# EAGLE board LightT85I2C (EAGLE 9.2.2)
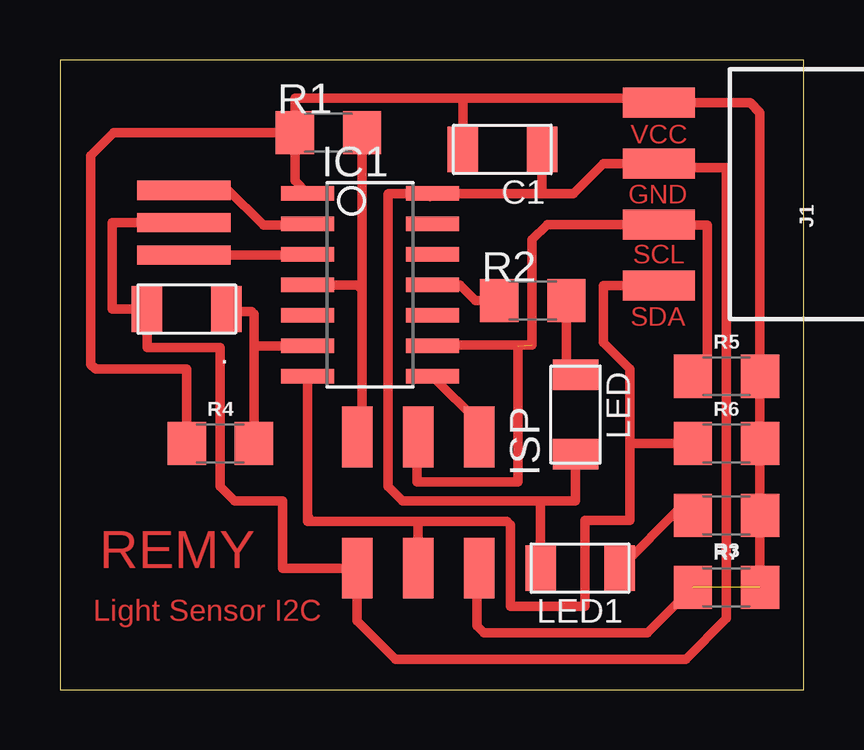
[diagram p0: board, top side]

Size 31 x 26.26 mm. Coordinates in mm from the lower left corner, seen from the top.
Outline: 0,0 31,0 31,26.26 0,26.26 0,0
Copper layers (1*16): Top 0.035mm / dielectric 1.5mm / Bottom 0.035mm
Design rules "default *": minimum track width 0.4mm, minimum drill 0.4mm, track to track 0.3mm, track to pad 0.3mm, pad to pad 0.3mm, via to via 6mil, smd to smd 0.3mm, copper to edge 40mil, drill to drill 6mil, minimum pad ring 10mil, minimum via ring 8mil, stop-mask expansion 4mil, vias tented up to drill 0mil, thermal gap 10mil

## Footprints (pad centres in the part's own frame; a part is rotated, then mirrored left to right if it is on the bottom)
LED1206FAB = smd 1.27 x 1.905: 1 -1.651,0; 2 1.651,0
C1206FAB = smd 1.27 x 1.905: 1 -1.651,0; 2 1.651,0
SOIC14 = smd 0.61 x 2.21: 1 -3.81,-2.603; 2 -2.54,-2.603; 3 -1.27,-2.603; 4 0,-2.603; 5 1.27,-2.603; 6 2.54,-2.603; 7 3.81,-2.603; 8 3.81,2.603; 9 2.54,2.603; 10 1.27,2.603; 11 0,2.603; 12 -1.27,2.603; 13 -2.54,2.603; 14 -3.81,2.603
2X03SMD = smd 2.54 x 1.27: 1 -2.54,2.54; 2 2.92,2.54; 3 -2.54,0; 4 2.92,0; 5 -2.54,-2.54; 6 2.92,-2.54
1X04_SMD_RA_FEMALE = smd 1.25 x 3: 1 -3.81,7.225; 2 -1.27,7.225; 3 1.27,7.225; 4 3.81,7.225
1206 = smd 1.6 x 1.8: 1 -1.4,0; 2 1.4,0
EFOBM = smd 0.8 x 3.9: 1 -1.35,0; 2 0,0; 3 1.35,0

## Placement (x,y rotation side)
.  Sensor  [LED1206FAB]  5.28,15.87 180 top
C1  10uF  [C1206FAB]  18.44,22.53 180 top
IC1  ATTINY44-SSU  [SOIC14]  12.93,16.88 270 top
ISP  AVRISPSMD  [2X03SMD]  14.93,7.99 270 top
J1  [1X04_SMD_RA_FEMALE]  32.18,20.67 90 top
LED  Red  [LED1206FAB]  21.5,11.48 270 top
LED1  Green  [LED1206FAB]  21.68,5.07 180 top
R1  10k  [1206]  11.19,23.23 0 top
R2  1000  [1206]  19.71,16.23 0 top
R3  449  [1206]  27.78,7.27 180 top
R4  49.9K  [1206]  6.68,10.27 0 top
R5  10k  [1206]  27.78,13.07 0 top
R6  10k  [1206]  27.78,10.27 0 top
R7  0  [1206]  27.78,4.27 0 top
XTAL1  20 Mhz  [EFOBM]  5.17,19.48 90 top

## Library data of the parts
. C1 IC1 ISP LED LED1 XTAL1 = fab
J1 = SparkFun-Connectors; PROD_ID: CONN-12382
R1-R7 = SparkFun-Resistors

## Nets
GND: ..2 C1.1 IC1.14 ISP.6 J1.3 LED1.2 LED.2 XTAL1.2
N$1: LED.1 R2.2
N$2: LED1.1 R3.2
PA0: IC1.13
PA1: IC1.12
PA2: IC1.11 R2.1
PA3: IC1.10
PA4: IC1.9 ISP.3 J1.2 R5.1
PA5: IC1.8 ISP.1
PA6: IC1.7 ISP.4 J1.1 R6.1
PA7: ..1 IC1.6 R4.2
PB0: IC1.2 XTAL1.3
PB1: IC1.3 XTAL1.1
PB2: IC1.5
PB3: IC1.4 ISP.5 R1.2
VCC: C1.2 IC1.1 ISP.2 J1.4 R1.1 R3.1 R4.1 R5.2 R6.2 R7.1 R7.2

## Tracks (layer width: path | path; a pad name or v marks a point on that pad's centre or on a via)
GND
  Top 0.4: 12.39,4.18 12.39,4.77 | 12.39,4.77 ISP.6 | 12.26,5.21 ISP.6 | 20.29,22.73 C1.1 20.1,20.69 | 15.42,20.57 IC1.14 | 12.38,4.77 12.39,4.77 | IC1.14 13.7,20.69 13.68,20.67 13.68,8.47 14.27,7.88 19.98,7.88 | 5.07,19.37 XTAL1.2 2.18,19.48 2.18,15.87 ..2 3.63,14.27 6.68,14.27 6.68,8.47 7.28,7.87 9.28,7.87 9.28,5.07 ISP.6 | LED.2 21.5,7.88 19.98,7.88 | IC1.14 20.1,20.69 | LED1.2 20.03,7.84 19.98,7.88 | 20.1,20.69 21.41,20.69 22.66,21.94 J1.3 25.13,21.77 27.78,21.77 27.78,2.97 26.08,1.27 13.98,1.27 12.39,2.87 ISP.6
N$1
  Top 0.4: R2.2 21.11,13.51 LED.1
N$2
  Top 0.4: LED1.1 25.88,7.62 25.88,6.97 26.08,6.97 R3.2
PA1
  Top 0.4: IC1.12 15.56,18.17
PA2
  Top 0.4: IC1.11 16.67,16.88 17.33,16.23 R2.1
PA4  (1 unrouted)
  Top 0.152: ISP.3
  Top 0.4: ISP.3 14.88,10.49 14.88,8.67 19.08,8.67 19.08,14.34 | R5.1 26.98,13.67 26.98,19.37 24.99,19.37 J1.2 20.31,19.4 19.68,18.77 19.68,14.37 15.57,14.37 IC1.9
PA5
  Top 0.4: ISP.1 17.47,11.14 IC1.8
PA6
  Top 0.4: IC1.7 10.33,7.23 | 10.33,7.23 10.33,7.03 14.93,7.03 | 10.33,7.23 10.38,7.17 | 14.93,7.03 14.93,7.02 ISP.4 | 23.76,10.07 23.76,10.27 R6.1 | 23.76,10.07 23.76,13.37 22.66,14.47 22.66,16.86 J1.1 | 23.76,10.07 23.76,7.07 21.88,7.07 21.88,3.47 18.78,3.47 18.78,6.87 18.63,7.03 14.93,7.03
PA7
  Top 0.4: 10.3,14.37 IC1.6 8.15,14.34 8.08,14.27 | 6.84,15.77 6.84,15.47 6.88,15.42 | 6.84,15.77 ..1 | R4.2 8.08,14.27 | 8.08,14.27 8.08,15.67 7.98,15.77 6.84,15.77
PB0
  Top 0.4: XTAL1.3 5.12,20.87 4.43,20.87 4.48,20.93 6.93,20.93 8.48,19.37 10.28,19.37 IC1.2
PB1
  Top 0.4: IC1.3 10.3,18.13 XTAL1.1
PB2
  Top 0.4: 10.3,15.64 IC1.5
PB3
  Top 0.4: ISP.5 12.59,10.74 12.59,16.67 | 10.44,16.77 IC1.4 12.38,16.88 12.59,16.67 | R1.2 12.59,16.67
VCC  (1 unrouted)
  Top 0.4: R1.1 9.79,21.23 IC1.1 | R1.1 9.79,24.67 16.79,24.67 | C1.2 16.79,24.67 | 9.73,23.17 R1.1 | ISP.2 17.38,4.99 17.38,2.67 17.68,2.37 24.48,2.37 R7.1 | R1.1 2.24,23.23 1.28,22.27 1.28,13.57 1.48,13.37 5.28,13.37 R4.1 | 16.79,24.67 25.15,24.67 J1.4 28.77,24.48 29.18,24.07 R5.2 R6.2 R3.1 | R3.1 29.08,7.17 | R3.1 R7.2 | R3.1 29.28,7.37

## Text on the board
Top: VCC | GND | SCL | SDA | REMY | Light Sensor I2C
